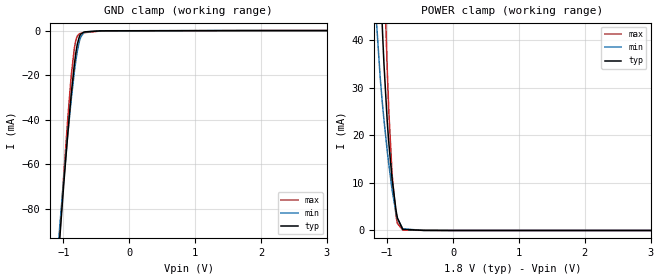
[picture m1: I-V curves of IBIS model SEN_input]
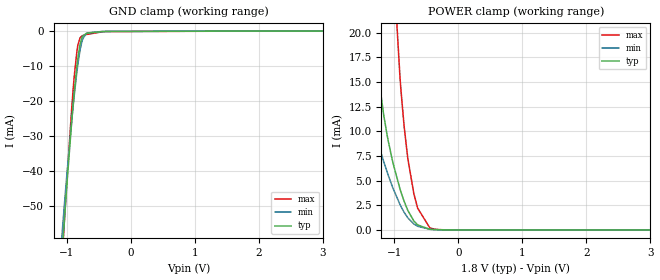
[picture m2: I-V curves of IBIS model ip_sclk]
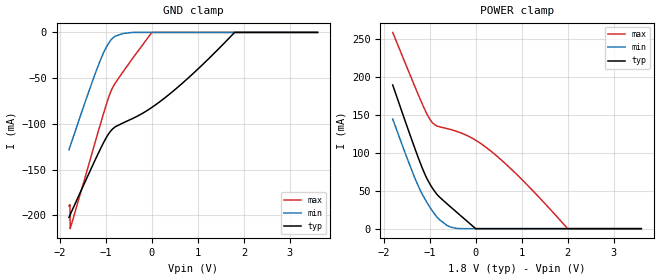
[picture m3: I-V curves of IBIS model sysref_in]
|Texas Instruments Incorporated
|ADC3669
[IBIS Ver]   4.1
[File name]   adc3669.ibs
[Date]   10/7/2022
[File Rev]   1.0
[Source]
| Texas Instruments Incorporated.
| Analog-eLab Design Center, HPA
| 12500 TI Blvd
| Dallas, TX -75243
[Notes]   Revision History:
| Rev 1.0: 06/25/2018
| - Initial version of the model
| - Model generated from simulations in SPECTRE
| - Warnings regarding combined Non-monotonicity of various models
|   have been reviewed and considered minor and can be ignored.
| - For diffin model, use suitable (100Ohms, 135Ohms, 200Ohms, 400Ohms) termination
|   externally, as internal termination is disabled.
| - C_comp although listed in numerical order of value are
|   obtained from varying PVT conditions. For PVT conditions for
|   each specific value refer the buffer description under
|   respective [Model]. IBIS model user is responsible for using
|   appropriate C_comp to simulate for Signal Integrity.
[Disclaimer]
| This model is designed as an aid for customers of Texas Instruments.
| TI and its licensors and suppliers make no warranties, either expressed
| or implied, with respect to this  model, including the warranties of
| merchantability or fitness for a particular purpose. The model is
| provided solely on an "as is" basis. The entire risk as to its quality
| and performance is with the customer.
| This model is subject to change without notice. Texas Instruments
| Incorporated is not responsible for updating this model.
[Copyright]
(C) Copyright 2018 Texas Instruments Incorporated.All rights reserved.
|  Component ADC3669 64 QFN package
|  Part # ADC3669
[Component]   ADC3669
[Manufacturer]  TI
[Package]   |64 QFN package
|   typ   min   max
R_pkg   0.60837   0.52897   0.78365
L_pkg   2.09208nH   1.78421nH   2.77432nH
C_pkg   0.17978pF   0.12083pF   0.27053pF
[Pin]  signal_name   model_name   R_pin   L_pin   C_pin
1   DGND   power   NA   NA   NA
2   DVDD12   power   NA   NA   NA
3   DOUT11P   Diff_op   NA   NA   NA
4   DOUT11M   Diff_op   NA   NA   NA
5   DOUT12P   Diff_op   NA   NA   NA
6   DOUT12M   Diff_op   NA   NA   NA
7   DOUT13P   Diff_op   NA   NA   NA
8   DOUT13M   Diff_op   NA   NA   NA
9   DOUT14P   Diff_op   NA   NA   NA
10   DOUT14M   Diff_op   NA   NA   NA
11   DOUT15P   Diff_op   NA   NA   NA
12   DOUT15M   Diff_op   NA   NA   NA
13   SCLK   ip_sclk   NA   NA   NA
14   SEN   SEN_input   NA   NA   NA
15   AVDD12   power   NA   NA   NA
16   AGND   power   NA   NA   NA
17   AVDD18   power   NA   NA   NA
18   AINP   nc   NA   NA   NA
19   AINM   nc   NA   NA   NA
20   AVDD18   power   NA   NA   NA
21   VCM   nc   NA   NA   NA
22   AVDD12   power   NA   NA   NA
23   CLKGND   power   NA   NA   NA
24   CLKP   ip_clk   NA   NA   NA
25   CLKM   ip_clk   NA   NA   NA
26   CLKGND   power   NA   NA   NA
27   GPIO0   sysref_in   NA   NA   NA
28   GPIO1   sysref_in   NA   NA   NA
29   AVDD18   power   NA   NA   NA
30   BINM   nc   NA   NA   NA
31   BINP   nc   NA   NA   NA
32   AVDD18   power   NA   NA   NA
33   AGND   power   NA   NA   NA
34   AVDD12   power   NA   NA   NA
35   RESET   SEN_input   NA   NA   NA
36   SDIO   sdata_io   NA   NA   NA
37   DOUT0/FCLKM   Diff_op   NA   NA   NA
38   DOUT0/FCLKP   Diff_op   NA   NA   NA
39   DOUT1M   Diff_op   NA   NA   NA
40   DOUT1P   Diff_op   NA   NA   NA
41   DOUT2M   Diff_op   NA   NA   NA
42   DOUT2P   Diff_op   NA   NA   NA
43   DOUT3M   Diff_op   NA   NA   NA
44   DOUT3P   Diff_op   NA   NA   NA
45   DOUT4M   Diff_op   NA   NA   NA
46   DOUT4P   Diff_op   NA   NA   NA
47   DVDD12   power   NA   NA   NA
48   DGND   power   NA   NA   NA
49   DOUT5P   Diff_op   NA   NA   NA
50   DOUT5M   Diff_op   NA   NA   NA
51   DOUT6P   Diff_op   NA   NA   NA
52   DOUT6M   Diff_op   NA   NA   NA
53   DOUT7P   Diff_op   NA   NA   NA
54   DOUT7M   Diff_op   NA   NA   NA
55   DCLKP   Diff_op   NA   NA   NA
56   DCLKM   Diff_op   NA   NA   NA
57   DGND   power   NA   NA   NA
58   DVDD18   power   NA   NA   NA
59   DOUT8M   Diff_op   NA   NA   NA
60   DOUT8P   Diff_op   NA   NA   NA
61   DOUT9M   Diff_op   NA   NA   NA
62   DOUT9P   Diff_op   NA   NA   NA
63   DOUT10M   Diff_op   NA   NA   NA
64   DOUT10P   Diff_op   NA   NA   NA
[Diff pin]  inv_pin  vdiff  tdelay_typ  tdelay_min  tdelay_max
3   4   0.0   0.0s   0.0s   0.0s
5   6   0.0   0.0s   0.0s   0.0s
7   8   0.0   0.0s   0.0s   0.0s
9   10   0.0   0.0s   0.0s   0.0s
11   12   0.0   0.0s   0.0s   0.0s
24   25   0.1   0.0s   0.0s   0.0s
38   37   0.0   0.0s   0.0s   0.0s
40   39   0.0   0.0s   0.0s   0.0s
42   41   0.0   0.0s   0.0s   0.0s
44   43   0.0   0.0s   0.0s   0.0s
46   45   0.0   0.0s   0.0s   0.0s
49   50   0.0   0.0s   0.0s   0.0s
51   52   0.0   0.0s   0.0s   0.0s
53   54   0.0   0.0s   0.0s   0.0s
55   56   0.0   0.0s   0.0s   0.0s
60   59   0.0   0.0s   0.0s   0.0s
62   61   0.0   0.0s   0.0s   0.0s
64   63   0.0   0.0s   0.0s   0.0s
| Models and submodels in the file (6): SEN_input (Input), ip_sclk (Input), sysref_in (Input), sdata_io (I/O), Diff_op (Output), ip_clk (Input)
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|   SEN_input Model
[Model]   SEN_input
Model_type   Input
Vinl = 0.4
Vinh = 1.3
|   typ   min   max
C_comp   1.373pF   1.281pF   1.464pF
| Where C_comp = 1.373pF at 1.8V, 27C and nominal process
| Where C_comp = 1.464pF at 1.75V, 105C and weak process
| Where C_comp = 1.281pF at 2V, -40C and strong process
[Voltage Range]   1.8   1.75   2
|Junction Temperature
[Temperature Range]   27   105   -40
[Power Clamp Reference]   1.8   1.75   2
[GND Clamp Reference]   0   0   0
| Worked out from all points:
|   GND clamp passes 1 mA (typ) near -0.71 V on its own axis
|   POWER clamp passes 1 mA (typ) near -0.79 V on its own axis
[GND Clamp]
|   Voltage   I(typ)   I(min)   I(max)
-1.8V     -431.8mA   -399.9mA   -451.9mA
-1.157V   -136.3mA   -125.7mA   -138.4mA
-1.055V   -92.71mA   -87.35mA   -91mA
-1.012V   -75.26mA   -72.18mA   -71.77mA
-936mV    -46.79mA   -47.22mA   -40.16mA
-876.6mV  -27.01mA   -29.47mA   -18.88mA
-833.4mV  -14.92mA   -18.24mA   -7.648mA
-811.8mV  -10.03mA   -13.42mA   -4.273mA
-757.8mV  -2.669mA   -4.79mA    -1.465mA
-666mV    -567.2uA   -580.7uA   -886.6uA
-444.6mV  -132.9uA   -102.5uA   -223.8uA
3.6V      0A         0A         0A
[POWER Clamp]
|   Voltage   I(typ)   I(min)   I(max)
-1.8V     450.2mA    350.1mA    527.5mA
-1.174V   83.67mA    46.03mA    124.1mA
-1.076V   43.49mA    27.25mA    69.6mA
-1.071V   41.7mA     26.43mA    66.81mA
-1.049V   35.09mA    23.29mA    55.98mA
-1.001V   23.24mA    16.92mA    34.41mA
-973.8mV  18.14mA    13.71mA    24.64mA
-925.2mV  10.77mA    8.544mA    11.75mA
-865.8mV  4.225mA    3.671mA    3.033mA
-844.2mV  2.611mA    2.434mA    1.482mA
-763.2mV  225.6uA    333.5uA    84.77uA
3.6V      0A         0A         0A
|   ip_sclk Model
[Model]   ip_sclk
Model_type   Input
Vinl = 0.4
Vinh = 1.3
|   typ   min   max
C_comp   0.3263pF   0.2868pF   0.3661pF
| Where C_comp = 0.3263pF at 1.8V, 27C and nominal process
| Where C_comp = 0.3661pF at 1.75V, 105C and weak process
| Where C_comp = 0.2868pF at 2V, -40C and strong process
[Voltage Range]   1.8   1.75   2
|Junction Temperature
[Temperature Range]   27   105   -40
[Power Clamp Reference]   1.8   1.75   2
[GND Clamp Reference]   0   0   0
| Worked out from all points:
|   GND clamp passes 1 mA (typ) near -0.72 V on its own axis
|   POWER clamp passes 1 mA (typ) near -0.70 V on its own axis
[GND Clamp]
|   Voltage   I(typ)   I(min)   I(max)
-1.8V     -285mA     -259mA     -304.4mA
-1.152V   -86.99mA   -77.78mA   -90.52mA
-1.06V    -60.99mA   -55.34mA   -61.81mA
-1.017V   -49.34mA   -45.52mA   -48.78mA
-919.8mV  -25.55mA   -25.44mA   -21.82mA
-898.2mV  -20.9mA    -21.4mA    -16.64mA
-838.8mV  -9.845mA   -11.49mA   -5.619mA
-790.2mV  -3.768mA   -5.389mA   -1.938mA
-763.2mV  -1.991mA   -3.128mA   -1.414mA
-693mV    -663uA     -692.3uA   -992.5uA
-342mV    -103.3uA   -86.91uA   -137.7uA
3.6V      0A         0A         0A
[POWER Clamp]
|   Voltage   I(typ)   I(min)   I(max)
-1.8V     82.98mA    30.3mA     184.2mA
-1.649V   58.42mA    21.28mA    150mA
-1.325V   20.75mA    10.53mA    80.63mA
-1.163V   11.64mA    6.932mA    50.07mA
-1.017V   6.768mA    4.218mA    27.5mA
-909mV    4.165mA    2.581mA    15.5mA
-844.2mV  2.907mA    1.793mA    10.51mA
-784.8mV  1.959mA    1.219mA    7.174mA
-633.6mV  513.9uA    371.5uA    2.216mA
-444.6mV  71.84uA    73.6uA     229.7uA
-331.2mV  27.83uA    31.13uA    55.37uA
3.6V      0A         0A         0A
|   sysref_diff_in Model
[Model]   sysref_in
Model_type   Input
Vinl = 0.4
Vinh = 1.3
|   typ   min   max
C_comp   0.50774pF   0.5054pF   0.59929pF
| Where C_comp = 0.5054pF at 1.8V, 27C and nominal process
| Where C_comp = 0.59929pF at 1.75V, 105C and weak process
| Where C_comp = 0.50774pF at 2V, -40C and strong process
[Voltage Range]   1.8   1.75   2
|Junction Temperature
[Temperature Range]   27   105   -40
[Power Clamp Reference]   1.8   1.75   2
[GND Clamp Reference]   0   0   0
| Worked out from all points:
|   POWER clamp passes 1 mA (typ) near -0.02 V on its own axis
[GND Clamp]
|   Voltage   I(typ)   I(min)   I(max)
-1.8V     -202.2mA   -128.4mA   -189.7mA
-1.778V   -199.7mA   -125.1mA   -188.3mA
-1.773V   -199.1mA   -124.3mA   -214.5mA
-1.195V   -135.6mA   -40.33mA   -113.8mA
-1.049V   -120.6mA   -22.34mA   -88.75mA
-914.4mV  -109.1mA   -10.1mA    -67.72mA
-806.4mV  -103.6mA   -4.444mA   -56.23mA
-622.8mV  -98.88mA   -1.277mA   -42.91mA
-1.8mV    -82.05mA   0A         -123.2uA
765mV     -51mA      0A         0A
1.796V    -101.5uA   0A         0A
3.6V      0A         0A         0A
[POWER Clamp]
|   Voltage   I(typ)   I(min)   I(max)
-1.8V     189.5mA    144.5mA    258.8mA
-1.298V   102.3mA    63.67mA    184.3mA
-1.087V   69.91mA    37.71mA    155mA
-995.4mV  59.19mA    28.59mA    144.4mA
-919.8mV  51.86mA    21.67mA    138.7mA
-784.8mV  41.74mA    11.89mA    134.3mA
-536.4mV  28.32mA    2.003mA    130.6mA
-1.8mV    182.1uA    0A         116.8mA
360mV     0A         0A         100.9mA
808.2mV   0A         0A         76.54mA
1.996V    0A         0A         260uA
3.6V      0A         0A         0A
